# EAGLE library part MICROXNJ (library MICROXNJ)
MICRO-USB-SMD_MICROXNJ Source: Datasheet
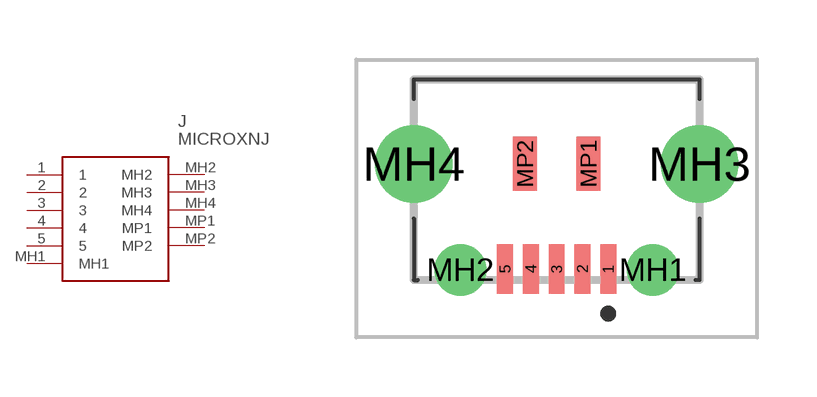
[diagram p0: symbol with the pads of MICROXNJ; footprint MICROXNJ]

Designator prefix J

## MICROXNJ (Description: MICRO-USB-SMD_MICROXNJ; Height: 2.425mm; Manufacturer_Name: Shou Han; Manufacturer_Part_Number: MICROXNJ)  [MICROXNJ]
1  1
2  2
3  3
4  4
5  5
MH1  MH1
MH2  MH2
MH3  MH3
MH4  MH4
MP1  MP1
MP2  MP2

## Footprint MICROXNJ (pad centres in mm)
MICROXNJ-1
smd 0.4 x 1.25: 1 1.3,-4.775; 2 0.65,-4.775; 3 0,-4.775; 4 -0.65,-4.775; 5 -1.3,-4.775
drill 0.7 pad 1.3: MH1 2.425,-4.8; MH2 -2.425,-4.8
drill 1.3 pad 1.9: MH3 3.6,-2.13; MH4 -3.6,-2.13
smd 0.6 x 1.35: MP1 0.8,-2.125; MP2 -0.8,-2.125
